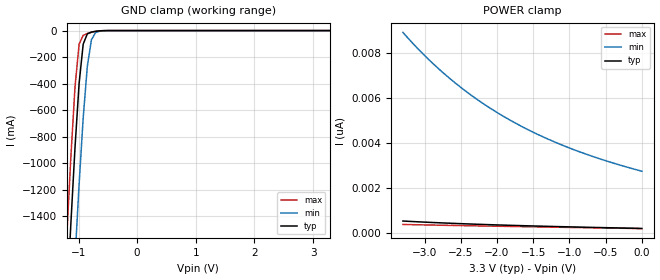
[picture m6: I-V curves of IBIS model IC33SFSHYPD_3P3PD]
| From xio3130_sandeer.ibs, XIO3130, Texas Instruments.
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|   5E-09S   0.66010mV   19.83000mV   14.01000uV
|   5.05E-09S   0.66010mV   16.93000mV   14.01000uV
|   5.1E-09S   0.66010mV   15.18000mV   14.01000uV
|   5.15E-09S   0.66010mV   13.67000mV   14.01000uV
|   5.2E-09S   0.66010mV   12.69000mV   14.01000uV
|   5.25E-09S   0.66010mV   11.82000mV   14.01000uV
|   5.3E-09S   0.66010mV   11.18000mV   14.01000uV
|   5.35E-09S   0.66010mV   10.58000mV   14.01000uV
|   5.4E-09S   0.66010mV   10.05000mV   14.01000uV
|   5.45E-09S   0.66010mV   9.54200mV   14.01000uV
|   5.5E-09S   0.66010mV   9.05200mV   14.01000uV
|   5.55E-09S   0.66010mV   8.56700mV   14.01000uV
|   5.6E-09S   0.66010mV   8.09100mV   14.01000uV
|   5.65E-09S   0.66010mV   7.61700mV   14.01000uV
|   5.7E-09S   0.66010mV   7.15900mV   14.01000uV
|   5.75E-09S   0.66010mV   6.70300mV   14.01000uV
|   5.8E-09S   0.66010mV   6.27300mV   14.01000uV
|   5.85E-09S   0.66010mV   5.84700mV   14.01000uV
|   5.9E-09S   0.66010mV   5.45300mV   14.01000uV
|   5.95E-09S   0.66010mV   5.06400mV   14.01000uV
|   6E-09S   0.66010mV   4.71000mV   14.01000uV
|   6.05E-09S   0.66010mV   4.36100mV   14.01000uV
|   6.1E-09S   0.66010mV   4.04700mV   14.01000uV
|   6.15E-09S   0.66010mV   3.74000mV   14.01000uV
|   6.2E-09S   0.66010mV   3.46500mV   14.01000uV
|   6.25E-09S   0.66010mV   3.19600mV   14.01000uV
|   6.3E-09S   0.66010mV   2.95800mV   14.01000uV
|   6.35E-09S   0.66010mV   2.72700mV   14.01000uV
|   6.4E-09S   0.66010mV   2.52300mV   14.01000uV
|   6.45E-09S   0.66010mV   2.32400mV   14.01000uV
|   6.5E-09S   0.66010mV   2.14900mV   14.01000uV
|   6.55E-09S   0.66010mV   1.97900mV   14.01000uV
|   6.6E-09S   0.66010mV   1.82900mV   14.01000uV
|   6.65E-09S   0.66010mV   1.68300mV   14.01000uV
|   6.7E-09S   0.66010mV   1.55000mV   14.01000uV
|   6.75E-09S   0.66010mV   1.42100mV   14.01000uV
|   6.8E-09S   0.66010mV   1.31100mV   14.01000uV
|   6.85E-09S   0.66010mV   1.20500mV   14.01000uV
|   6.9E-09S   0.66010mV   1.10800mV   14.01000uV
|   6.95E-09S   0.66010mV   1.02600mV   14.01000uV
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[Model]   IC33SFSHYPD_3P3PD
Model_type   Input
Polarity   Non-Inverting
Vinl =   0.9900V
Vinh =   2.3100V
C_comp   2.0300pF   2.1210pF   2.0450pF
[Model Spec]
|   typ   min   max
Vinh   2.31V   2.10V   2.52V
Vinl   0.99V   0.90V   1.08V
[Temperature Range]   25.0000   0.1250k   -40.0000
[Voltage Range]   3.3000V   3.0000V   3.6000V
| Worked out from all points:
|   GND clamp passes 1 mA (typ) near -0.59 V on its own axis
| (Vdd votage range)   1.50V   1.35V   1.65V
| (Process strength)   nominal   weak   strong
[GND_clamp]
| voltage   I(typ)   I(min)   I(max)
-3.3V     -22.44A    -23.23A    -22.01A
-1.2V     -2.062A    -2.938A    -1.55A
-1.13V    -1.453A    -2.319A    -952.1mA
-1.06V    -884.3mA   -1.722A    -427mA
-990mV    -399.1mA   -1.159A    -102.3mA
-920mV    -102mA     -657.3mA   -35.66mA
-850mV    -24.66mA   -270.7mA   -22.38mA
-780mV    -11.46mA   -70.03mA   -12.94mA
-710mV    -5.644mA   -15.31mA   -5.841mA
-640mV    -2.142mA   -4.307mA   -1.755mA
3.28V     193.3pA    3.002nA    169pA
[POWER_clamp]
| voltage   I(typ)   I(min)   I(max)
-3.3V     528.5pA    8.938nA    374.6pA
-3V       479pA      7.907nA    354.7pA
-2.85V    456.8pA    7.444nA    345.7pA
-2.65V    429.6pA    6.877nA    333.3pA
-2.3V     386.9pA    6.006nA    313pA
-2.1V     365.3pA    5.571nA    302.1pA
-1.9V     344.8pA    5.175nA    290.8pA
-1.5V     308.2pA    4.487nA    269.3pA
-1.05V    271.5pA    3.848nA    245.4pA
-550mV    235pA      3.27nA     219.2pA
0V        195.4pA    2.748nA    187.9pA
